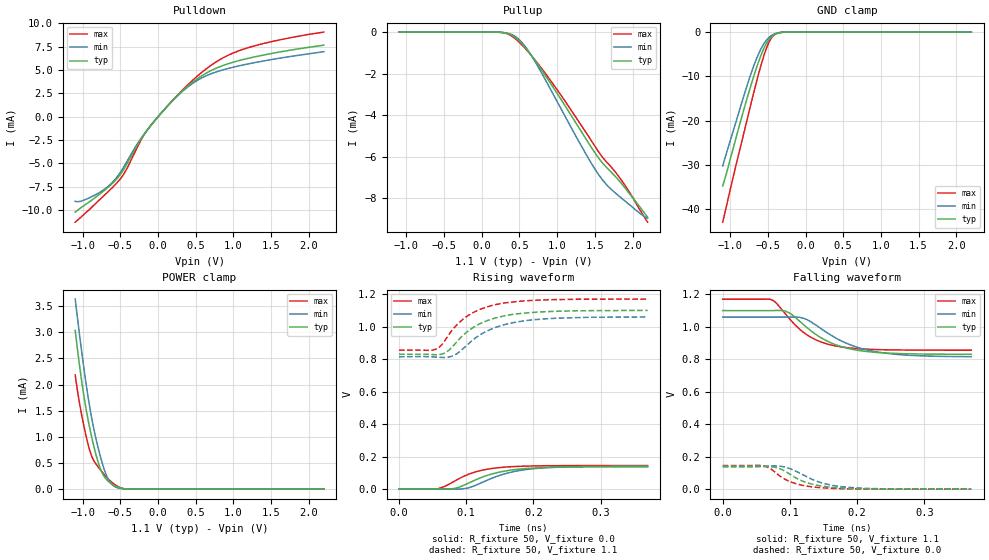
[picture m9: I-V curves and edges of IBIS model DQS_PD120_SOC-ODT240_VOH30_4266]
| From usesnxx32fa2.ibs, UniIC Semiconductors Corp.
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| DQS_PD120_SOC-ODT240_VOH30_4266
| (120 Ohm Pulldown, 240 Ohm System ODT Setting, VOH=VDDQ/3.0, 3200-4266Mbps)
[Model]   DQS_PD120_SOC-ODT240_VOH30_4266
Model_type   I/O
Vinl = 123.333mV
Vinh = 243.333mV
Vmeas = 183.333mV
Vref = 0.0mV
Cref = 0.0pF
Rref = 240.000Ohm
|   typ   min   max
|C_comp   0.849pF   0.799pF   0.899pF
C_comp_pullup   0.4245pF   0.3995pF   0.4495pF
C_comp_pulldown   0.4245pF   0.3995pF   0.4495pF
| Note: C_comp changes when the ODT circuit is enabled.
[Model Spec]
| Input threshold voltage corners
Vinl   0.1233V   0.1167V   0.1350V
Vinh   0.2433V   0.2367V   0.2550V
| Measurement voltage corners
Vmeas   0.1833V   0.1767V   0.1950V
| Timing spec test load voltage corners
Vref   0.0000V   0.0000V   0.0000V
| Dynamic Overshoot Parameters from LPDDR4 Specification
D_overshoot_ampl_h   0.30   NA   NA
D_overshoot_ampl_l   0.30   NA   NA
D_overshoot_area_h   0.1n   NA   NA
D_overshoot_area_l   0.1n   NA   NA
[Voltage Range]   1.1000V   1.0600V   1.1700V
[Pullup Reference]   1.1000V   1.0600V   1.1700V
| Junction Temperature (Ambient temp is 35C typ 95C min -40C max)
[Temperature Range]   50.0   110.0   -40.0
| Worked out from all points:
|   slope of the pulldown table from 0 to 0.165 V, typ, clamps not added: 110 ohm
|   slope of the pullup table from 0 to 0.165 V, typ, clamps not added: 79 kohm
|   GND clamp passes 1 mA (typ) near -0.45 V on its own axis
|   POWER clamp passes 1 mA (typ) near -0.88 V on its own axis
|   rising waveform, R_fixture 50, V_fixture 0.0: 20-80 % time 57.1ps typ, 59.6ps min, 49.5ps max; typ from 0 V to 0.137 V
|   falling waveform, R_fixture 50, V_fixture 1.1: 20-80 % time 60.4ps typ, 69.4ps min, 51.2ps max; typ from 1.1 V to 0.831 V
|   rising waveform, R_fixture 50, V_fixture 1.1: 20-80 % time 56.5ps typ, 60.7ps min, 52.1ps max; typ from 0.83 V to 1.1 V
|   falling waveform, R_fixture 50, V_fixture 0.0: 20-80 % time 43.2ps typ, 49.6ps min, 38.7ps max; typ from 0.137 V to 0 V
[Pulldown]
|   Voltage   I(typ)   I(min)   I(max)
-1.1V     -10.24mA   -9.066mA   -11.32mA
-911.9mV  -9.128mA   -8.702mA   -9.957mA
-638mV    -7.389mA   -7.297mA   -7.849mA
-463.1mV  -5.75mA    -5.483mA   -6.247mA
-192.5mV  -1.976mA   -1.949mA   -2.04mA
45.1mV    420.7uA    419.5uA    417.6uA
355.3mV   2.997mA    2.933mA    3.1mA
625.9mV   4.603mA    4.336mA    5.043mA
860.2mV   5.481mA    5.016mA    6.299mA
1.137V    6.142mA    5.559mA    7.248mA
1.629V    6.957mA    6.293mA    8.262mA
2.2V      7.669mA    6.972mA    9.07mA
[GND Clamp]
|   Voltage   I(typ)   I(min)   I(max)
-1.1V     -34.74mA   -30.21mA   -42.91mA
-948.2mV  -25.43mA   -21.63mA   -31.79mA
-796.4mV  -16.11mA   -13.14mA   -21.19mA
-720.5mV  -11.75mA   -9.185mA   -15.87mA
-664.4mV  -8.736mA   -6.578mA   -12.07mA
-591.8mV  -5.255mA   -3.789mA   -7.492mA
-522.5mV  -2.665mA   -1.905mA   -3.811mA
-466.4mV  -1.297mA   -944.5uA   -1.691mA
-413.6mV  -566.2uA   -418.1uA   -620.7uA
-347.6mV  -154.9uA   -118uA     -135.5uA
-242mV    -10.28uA   -9.19uA    -5.672uA
2.2V      0A         0A         0A
[Pullup]
|   Voltage   I(typ)   I(min)   I(max)
-1.1V     1.046uA    1.612uA    471.2nA
236.5mV   -8.718uA   -8.625uA   -9.172uA
355.3mV   -78.49uA   -64.06uA   -108.1uA
457.6mV   -294.4uA   -245.6uA   -359.9uA
566.5mV   -699.5uA   -652.6uA   -750.4uA
695.2mV   -1.311mA   -1.351mA   -1.297mA
1.052V    -3.249mA   -3.698mA   -3.047mA
1.375V    -5.105mA   -5.833mA   -4.795mA
1.553V    -6.084mA   -6.882mA   -5.782mA
1.675V    -6.593mA   -7.426mA   -6.335mA
1.887V    -7.444mA   -8.098mA   -7.311mA
2.2V      -8.92mA    -8.97mA    -9.16mA
[POWER Clamp]
|   Voltage   I(typ)   I(min)   I(max)
-1.1V     3.033mA    3.633mA    2.184mA
-1.041V   2.345mA    2.929mA    1.625mA
-981.2mV  1.753mA    2.275mA    1.183mA
-911.9mV  1.2mA      1.611mA    764.5uA
-852.5mV  818.2uA    1.148mA    543.7uA
-779.9mV  447.8uA    701.4uA    396.3uA
-713.9mV  239.2uA    373.1uA    278.6uA
-654.5mV  142.6uA    170.4uA    185.9uA
-598.4mV  83.66uA    71.95uA    113uA
-489.5mV  17.76uA    10.87uA    22.47uA
-374mV    1.392uA    1.001uA    1.127uA
2.2V      0A         0A         0A
[Ramp]
|   typ   min   max
| 20% - 80%
dV/dt_r   82.32m/57.11p   84.05m/59.55p   87.11m/49.55p
dV/dt_f   161.59m/60.34p   146.48m/69.52p   188.39m/51.18p
| 25% - 75%
|dV/dt_r   68.60m/45.49p   70.04m/47.42p   72.59m/39.29p
|dV/dt_f   134.65m/48.01p   122.06m/55.37p   156.99m/40.66p
R_load = 50
[Rising Waveform]
R_fixture = 50
V_fixture = 0.0
|   Time   V(typ)   V(min)   V(max)
0s        149.4uV    121uV      112.3uV
57ps      90.13uV    184.4uV    2.263mV
68ps      -135.6uV   -21.87uV   16.9mV
81ps      3.256mV    -45.93uV   45.59mV
105ps     40.06mV    9.983mV    93.87mV
127ps     78.49mV    47.36mV    119.2mV
150ps     105.2mV    84.9mV     132.9mV
183ps     124.8mV    117mV      141mV
222ps     133.4mV    132.7mV    144.1mV
370ps     137.3mV    140.2mV    145.3mV
[Falling Waveform]
R_fixture   = 50
V_fixture   = 1.1
V_fixture_min = 1.06
V_fixture_max = 1.17
|   Time   V(typ)   V(min)   V(max)
0s        1.1V       1.06V      1.17V
72ps      1.1V       1.06V      1.168V
81ps      1.101V     1.06V      1.141V
94ps      1.096V     1.06V      1.077V
121ps     1.011V     1.052V     963.6mV
139ps     952mV      1.01V      919.1mV
164ps     896.4mV    941.3mV    885.4mV
195ps     859.9mV    881.2mV    867.2mV
232ps     841.4mV    843.7mV    859.5mV
370ps     830.7mV    815.9mV    856mV
[Rising Waveform]
R_fixture   = 50
V_fixture   = 1.1
V_fixture_min = 1.06
V_fixture_max = 1.17
|   Time   V(typ)   V(min)   V(max)
0s        830.4mV    814.6mV    855.9mV
56ps      827.3mV    811.9mV    863.6mV
72ps      848mV      811.5mV    937.5mV
83ps      892.5mV    825.9mV    997.4mV
95ps      945.6mV    862.8mV    1.045V
119ps     1.015V     945.4mV    1.104V
146ps     1.056V     998.7mV    1.138V
175ps     1.079V     1.029V     1.155V
219ps     1.093V     1.049V     1.165V
370ps     1.1V       1.06V      1.17V
[Falling Waveform]
R_fixture = 50
V_fixture = 0.0
|   Time   V(typ)   V(min)   V(max)
0s        137.5mV    140.4mV    145.3mV
58ps      139.2mV    141.1mV    145.3mV
68ps      139.4mV    142.8mV    133.3mV
77ps      135.5mV    143.6mV    107.7mV
102ps     86.43mV    123.3mV    43.64mV
120ps     47.77mV    86.95mV    22.86mV
139ps     25.34mV    50.33mV    11.55mV
165ps     10.71mV    22.44mV    4.606mV
201ps     3.368mV    7.364mV    1.351mV
370ps     231.2uV    263.9uV    135.4uV
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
